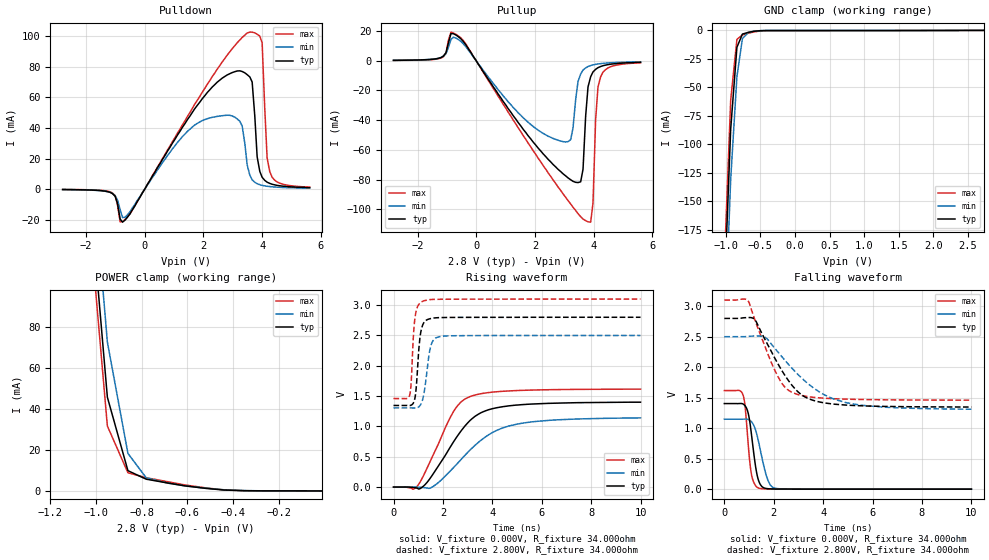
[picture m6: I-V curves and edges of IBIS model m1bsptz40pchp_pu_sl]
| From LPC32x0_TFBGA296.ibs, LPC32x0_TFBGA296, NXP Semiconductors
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| |   Rev 0.20 IBIS Model Design Automation Generation   |
| |   N O N - S I L I C O N   C O R R E L A T E D   |
| |   This IBIS [Model] is pre-Beta tactical support   |
| |  Note: this IBIS [Model] contains clamp curves generated   |
| |   through simulation which should not be relied upon   |
| mem1bsptz40pchp
|   Bidirectional Pad 2.8
|   3state Output
|   Plain Input
|   1ns Slew Rate control
|   CMOS
| Pull Up Mode (p1=0, p2=0)
[Model]   m1bsptz40pchp_pu_sl | of mem1bsptz40pchp
Model_type   I/O
Polarity   Non-Inverting
Enable   Active-Low
|  Reciever Thresholds
Vinl   = 0.36V
Vinh   = 0.84V
| AC Test Load Conditions
Vref   = 0
Cref   = 1.2e-11
Rref   = 1000000000
Vmeas   = 0.6
| [Process Range]   typical   min   max
| C_comp edge width   400.000ps   400.000ps   400.000ps
| C_comp Tstrobe   40.000fs   40.000fs   40.000fs
C_comp   2.019pF   1.948pF   2.108pF
[Temperature Range]   25   125   -40
[Voltage Range]   2.80V   2.50V   3.10V
[GND Clamp Reference]   0.00V   0.00V   0.00V
[Pulldown Reference]   0.00V   0.00V   0.00V
[POWER Clamp Reference]   2.80V   2.50V   3.10V
[Pullup Reference]   2.80V   2.50V   3.10V
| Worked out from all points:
|   slope of the pulldown table from 0 to 0.42 V, typ, clamps not added: 30.8 ohm
|   slope of the pullup table from 0 to 0.42 V, typ, clamps not added: 32.9 ohm
|   GND clamp passes 1 mA (typ) near -0.61 V on its own axis
|   POWER clamp passes 1 mA (typ) near -0.49 V on its own axis
|   rising waveform, V_fixture 0.000V, R_fixture 34.000ohm: 20-80 % time 1.45ns typ, 1.86ns min, 1.13ns max; typ from 0.001 V to 1.4 V
|   falling waveform, V_fixture 0.000V, R_fixture 34.000ohm: 20-80 % time 280ps typ, 393ps min, 212ps max; typ from 1.4 V to 0.001 V
|   rising waveform, V_fixture 2.800V, R_fixture 34.000ohm: 20-80 % time 167ps typ, 239ps min, 140ps max; typ from 1.35 V to 2.8 V
|   falling waveform, V_fixture 2.800V, R_fixture 34.000ohm: 20-80 % time 1.3ns typ, 1.9ns min, 1.01ns max; typ from 2.8 V to 1.35 V
[GND Clamp]
| ref voltage   0.00V   0.00V   0.00V
|   Voltage   I(typ)   I(min)   I(max)
-2.8V     -3.643A    -3.653A    -3.644A
-1.01V    -211.8mA   -255.9mA   -186.6mA
-930mV    -86.61mA   -130.6mA   -61.25mA
-840mV    -14.85mA   -40.65mA   -7.873mA
-760mV    -3.232mA   -7.1mA     -3.891mA
-670mV    -1.663mA   -1.71mA    -2.461mA
-500mV    -316uA     -247.5uA   -559.8uA
2.73V     -11.67uA   31.94uA    -74.22uA
[Power Clamp]   | Vtable = Vcc - Vpad
| ref voltage   2.80V   2.50V   3.10V
|   Voltage   I(typ)   I(min)   I(max)
-2.82V    3.531A     3.518A     3.546A
-1.03V    149.7mA    178.4mA    134.4mA
-950mV    45.72mA    72.62mA    31.66mA
-860mV    9.875mA    18.31mA    8.866mA
-780mV    5.725mA    6.415mA    6.434mA
-690mV    3.961mA    3.875mA    4.58mA
-610mV    2.472mA    2.439mA    2.908mA
-440mV    442.3uA    569.4uA    500uA
-270mV    46.38uA    47.88uA    58.33uA
-10mV     1.584uA    1.118uA    2.104uA
[Pulldown]
| ref voltage   0.00V   0.00V   0.00V
|   Voltage   I(typ)   I(min)   I(max)
-2.8V     -319.6uA   -345.8uA   -253.3uA
-1.18V    -2.161mA   -2.188mA   -1.788mA
-670mV    -20.27mA   -18.52mA   -19.89mA
2.13V     63.2mA     46.08mA    68.58mA
3.24V     77.42mA    44.42mA    97.59mA
3.58V     73.44mA    9.097mA    102.8mA
3.66V     70.11mA    6.079mA    102.8mA
3.83V     21.16mA    3.502mA    101.4mA
4V        7.734mA    2.421mA    95.8mA
4.17V     4.509mA    1.835mA    20.44mA
4.26V     3.717mA    1.634mA    11.39mA
5.62V     949.5uA    582uA      1.265mA
[Pullup]   | Vtable = Vcc - Vpad
| ref voltage   2.80V   2.50V   3.10V
|   Voltage   I(typ)   I(min)   I(max)
-2.82V    285.4uA    305.9uA    228.1uA
-520mV    14.74mA    12.98mA    15.34mA
2.79V     -73.11mA   -53.54mA   -85.02mA
3.22V     -80.14mA   -53.09mA   -96.45mA
3.47V     -82.02mA   -13.95mA   -103mA
3.64V     -73.04mA   -6.264mA   -106.6mA
3.81V     -17.62mA   -3.881mA   -108.4mA
3.9V      -10.77mA   -3.241mA   -108.7mA
3.98V     -7.53mA    -2.776mA   -95.86mA
4.07V     -5.77mA    -2.424mA   -39.5mA
4.24V     -3.896mA   -1.928mA   -10.84mA
5.6V      -1.048mA   -714.3uA   -1.374mA
[Ramp]
R_load   = 34.000ohm
|   dV/dt(typ)   dV/dt(min)   dV/dt(max)
dV/dt_r   970.359mV/1.295ns   805.778mV/1.655ns   1.109V/1.030ns
dV/dt_f   1.000V/1.130ns   838.007mV/1.640ns   1.123V/890.000ps
[Rising Waveform]  | cubic spline decimation from 2001 points
V_fixture   = 0.000V
R_fixture   = 34.000ohm
|   Time   V(typ)   V(min)   V(max)
0s        719.9uV    560uV      1.036mV
780ps     -5.169mV   786.7uV    -33.71mV
975ps     -20.9mV    -1.364mV   23.04mV
1.54ns    178.6mV    -5.235mV   472.5mV
2.42ns    739.8mV    317.6mV    1.239V
2.74ns    928.8mV    457.9mV    1.406V
3.1ns     1.099V     611.7mV    1.492V
3.985ns   1.291V     895.2mV    1.565V
4.935ns   1.351V     1.033V     1.591V
10ns      1.4V       1.141V     1.615V
[Falling Waveform]  | cubic spline decimation from 2001 points
V_fixture   = 0.000V
R_fixture   = 34.000ohm
|   Time   V(typ)   V(min)   V(max)
0s        1.404V     1.148V     1.617V
750ps     1.398V     1.148V     1.55V
845ps     1.364V     1.149V     1.332V
970ps     1.236V     1.142V     712.1mV
1.08ns    952.4mV    1.112V     283.2mV
1.255ns   394.5mV    980.3mV    63.73mV
1.37ns    160.7mV    804.4mV    21.35mV
1.735ns   9.505mV    178.3mV    3.955mV
2.055ns   3.246mV    15.88mV    2.661mV
10ns      729.5uV    574.7uV    1.045mV
[Rising Waveform]  | cubic spline decimation from 2001 points
V_fixture   = 2.800V
V_fixture_min = 2.500V
V_fixture_max = 3.100V
R_fixture   = 34.000ohm
|   Time   V(typ)   V(min)   V(max)
0s        1.346V     1.306V     1.46V
660ps     1.345V     1.306V     1.525V
720ps     1.352V     1.306V     1.758V
825ps     1.404V     1.304V     2.608V
910ps     1.598V     1.305V     2.888V
1.07ns    2.46V      1.343V     3.034V
1.215ns   2.702V     1.505V     3.069V
1.505ns   2.778V     2.32V      3.092V
1.805ns   2.793V     2.474V     3.096V
10ns      2.8V       2.5V       3.1V
[Falling Waveform]  | cubic spline decimation from 2001 points
V_fixture   = 2.800V
V_fixture_min = 2.500V
V_fixture_max = 3.100V
R_fixture   = 34.000ohm
|   Time   V(typ)   V(min)   V(max)
0s        2.8V       2.5V       3.1V
965ps     2.814V     2.505V     3.084V
1.27ns    2.76V      2.512V     2.738V
1.67ns    2.434V     2.483V     2.312V
2.085ns   2.116V     2.289V     1.913V
2.42ns    1.885V     2.129V     1.687V
2.78ns    1.683V     1.964V     1.581V
3.525ns   1.466V     1.685V     1.51V
4.965ns   1.378V     1.416V     1.476V
10ns      1.347V     1.312V     1.46V
